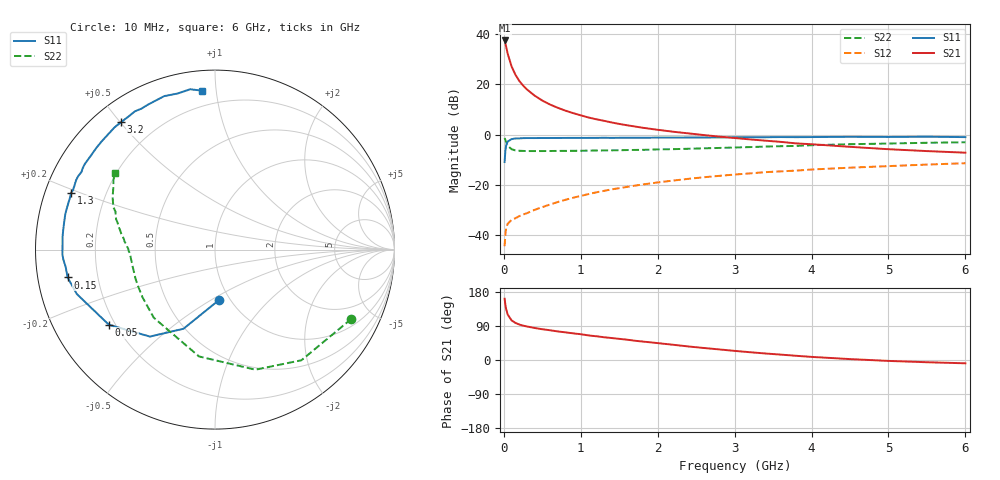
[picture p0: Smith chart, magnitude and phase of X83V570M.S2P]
! SIEMENS Small Signal Semiconductors
! BFP136W
! Si NPN RF Bipolar Junction Transistor in SOT343
! VCE = 3.5 V  IC = 70 mA
! Common Emitter S-Parameters:  September  1994
# GHz  S  MA  R  50
!  f  S11  S21  S12  S22
! GHz  MAG  ANG  MAG  ANG  MAG  ANG  MAG  ANG
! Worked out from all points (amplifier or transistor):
!   40 points, 10 MHz to 6 GHz, reference 50 ohm
!   highest |S21| = 37.4 dB at 10 MHz (marker M1)
!   |S21| within 3 dB of that: start of sweep to 33.61 MHz
!   unconditionally stable (mu >= 1): 577.5 MHz to 2.91 GHz
!   at 200 MHz: K = 0.62, MSG = 26.9 dB, |S12| = -32.5 dB
!   at 1.5 GHz: K = 1.11, MAG = 10.8 dB, |S12| = -21.4 dB
!   at 6 GHz: K = 0.96, MSG = 2.1 dB, |S12| = -11.4 dB
!   S11 on the Smith chart (normalised r, x): 10 MHz: 0.88, -0.54; 50 MHz: 0.18, -0.31; 150 MHz: 0.09, -0.09; 1.3 GHz: 0.08, +0.19; 3.2 GHz: 0.08, +0.50; 6 GHz: 0.11, +0.92
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0.01  0.2833 -85.9  74.46 161.7  0.006 71.0  0.8518 -27.0
0.02  0.4745 -111.7  65.17 146.0  0.0103 59.0  0.7822 -52.0
0.03  0.6052 -126.8  55.83 134.5  0.0136 51.0  0.706 -71.4
0.05  0.7245 -144.7  40.63 120.0  0.0167 39.2  0.6019 -98.5
0.1  0.8088 -162.2  22.76 104.7  0.02 34.3  0.5102 -132.0
0.15  0.8359 -169.3  15.54 97.9  0.0216 35.9  0.4834 -146.7
0.2  0.8372 -173.2  11.7 93.7  0.0237 37.7  0.4748 -154.7
0.25  0.8471 -176.4  9.439 90.7  0.0256 40.8  0.4718 -159.8
0.3  0.8508 -178.3  7.895 88.5  0.0272 43.5  0.4688 -163.2
0.4  0.8498 177.7  5.946 84.5  0.0317 47.4  0.4684 -167.8
0.5  0.8522 175.1  4.741 81.2  0.0359 51.0  0.4686 -170.8
0.6  0.8526 172.9  3.955 78.5  0.0405 53.6  0.4701 -172.7
0.7  0.8538 170.1  3.408 75.4  0.0453 55.9  0.4715 -174.1
0.9  0.8575 166.6  2.668 70.3  0.0552 57.9  0.4741 -176.7
1.1  0.8574 162.3  2.182 64.9  0.0652 59.0  0.4781 -178.4
1.3  0.8617 158.5  1.877 60.1  0.0756 59.4  0.4825 -180.0
1.7  0.8654 151.8  1.447 50.9  0.0959 57.9  0.4934 177.0
2.2  0.8672 143.2  1.137 40.2  0.1212 54.9  0.5111 173.4
3.2  0.8822 126.3  0.799 20.5  0.1686 46.0  0.5623 164.7
4.5  0.9007 108.3  0.569 2.4  0.2189 33.9  0.6416 152.8
5.5  0.904 98.8  0.468 -5.9  0.2522 26.0  0.6851 145.7
6  0.8881 94.6  0.435 -8.7  0.2687 21.7  0.7017 142.6
